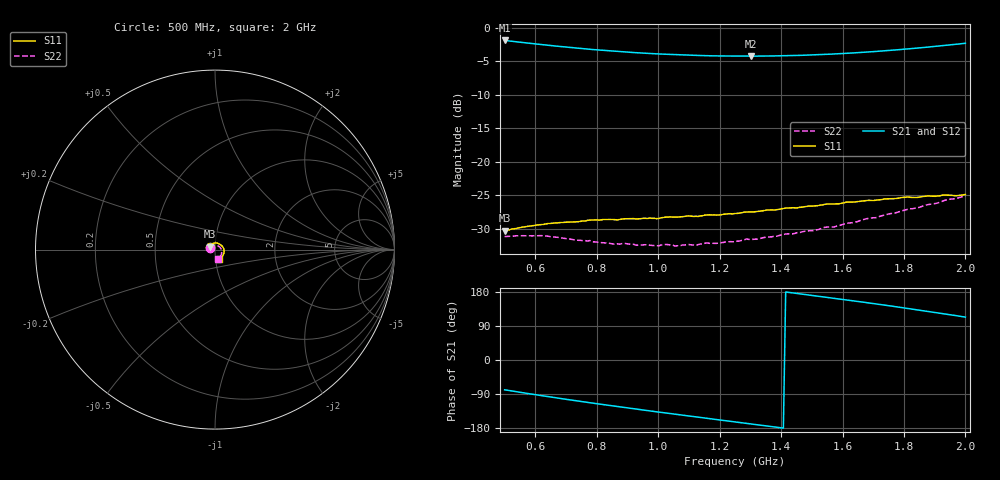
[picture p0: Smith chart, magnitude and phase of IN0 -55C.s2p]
!Agilent Technologies,E8363B,SG43030131,A.07.50.48
!Agilent E8363B: A.07.50.48
!Date: Friday, October 17, 2025 03:31:55
!Correction: S11(Full 2 Port(1,2))
!S21(Full 2 Port(1,2))
!S12(Full 2 Port(1,2))
!S22(Full 2 Port(1,2))
!S2P File: Measurements: S11, S21, S12, S22:
# Hz S  dB  R 50
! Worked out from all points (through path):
!   201 points, 500 MHz to 2 GHz, reference 50 ohm
!   highest |S21| = -1.92 dB at 500 MHz (marker M1); lowest = -4.3 dB at 1.302 GHz (marker M2)
!   group delay of S21, straight-line fit = 301 ps
!   lowest |S11| = -30.2 dB at 500 MHz (marker M3), VSWR 1.06, Z = 47.4 + j1.51 ohm
!   |S11| at or under -10 dB: start of sweep to end of sweep
!   |S22| runs from -32.5 to -25.0 dB; largest |S21 - S12| = 0.0015
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5e8  -30.22 148.8  -1.92 -78.6  -1.93 -78.6  -31.12 156.8
5.675e8  -29.65 134.4  -2.27 -87.4  -2.28 -87.5  -31.00 145.0
6.275e8  -29.30 123.3  -2.57 -95.0  -2.58 -95.0  -31.01 136.3
7.55e8  -28.79 101.3  -3.14 -110.1  -3.16 -110.2  -31.74 119.8
8.675e8  -28.63 85.4  -3.56 -122.9  -3.57 -122.9  -32.18 105.7
9.05e8  -28.44 80.1  -3.68 -127.0  -3.68 -127.0  -32.22 100.7
1.0025e9  -28.41 68.3  -3.93 -137.5  -3.94 -137.5  -32.48 90.6
1.025e9  -28.22 65.4  -3.98 -139.9  -3.99 -139.9  -32.28 88.0
1.055e9  -28.21 62.0  -4.04 -143.1  -4.05 -143.1  -32.54 84.2
1.1e9  -28.04 56.9  -4.12 -147.8  -4.12 -147.8  -32.30 78.3
1.1225e9  -28.10 54.3  -4.14 -150.1  -4.16 -150.2  -32.43 76.3
1.16e9  -27.90 50.1  -4.19 -154.1  -4.20 -154.0  -32.05 71.6
1.25e9  -27.68 39.7  -4.25 -163.4  -4.26 -163.4  -31.88 59.4
1.2875e9  -27.46 35.8  -4.25 -167.2  -4.26 -167.3  -31.47 54.4
1.3025e9  -27.43 33.8  -4.26 -168.8  -4.27 -168.8  -31.54 51.9
1.415e9  -26.87 21.9  -4.19 179.5  -4.20 179.5  -30.74 35.3
1.505e9  -26.57 11.5  -4.07 170.1  -4.08 170.1  -30.22 20.7
1.6325e9  -25.98 -4.1  -3.79 156.4  -3.79 156.4  -29.04 -2.4
1.7525e9  -25.49 -20.6  -3.41 143.1  -3.41 143.0  -27.73 -24.6
1.8275e9  -25.29 -31.9  -3.12 134.4  -3.13 134.4  -26.97 -39.1
1.8875e9  -25.10 -42.4  -2.87 127.3  -2.87 127.3  -26.29 -51.0
2e9  -24.85 -64.2  -2.34 113.1  -2.35 113.1  -25.03 -74.1
